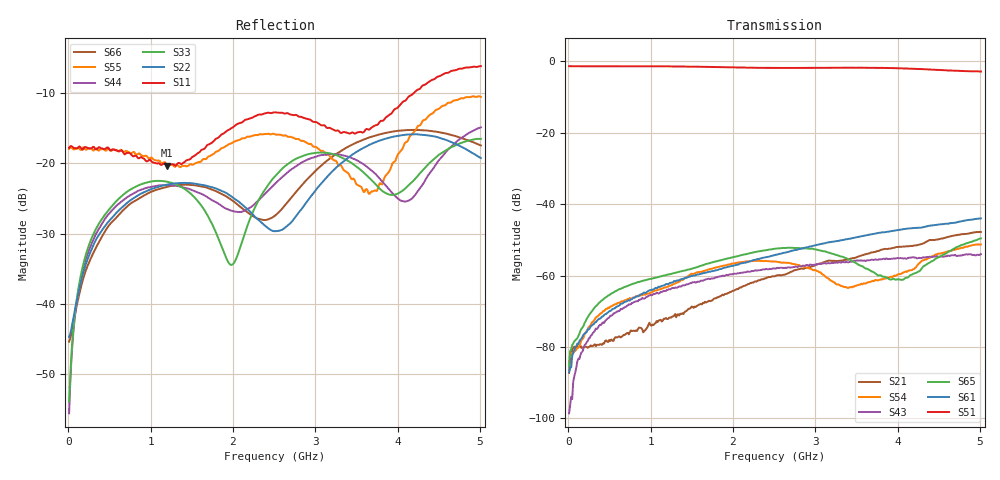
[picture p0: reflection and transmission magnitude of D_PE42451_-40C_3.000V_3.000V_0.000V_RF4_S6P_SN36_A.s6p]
! Device ID: PE42451
! Serial: 36
! Insertion: A
! Temp: -40C
! VDD: 3.000
! Control_Hi: 100.000
! Control_Lo: 0.000
! Logic State: RF4
! Port 1: RFC
! Port 2: RF1
! Port 3: RF2
! Port 4: RF3
! Port 5: RF4
! Port 6: RF5
! V1 = 0.00
! V2 = 0.00
! V3 = 3.00
! V4 = 0.00
! IDD: 1.326950e-05
#  Hz  S  RI  R  50
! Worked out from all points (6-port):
!   401 points, 10 MHz to 5.01 GHz, reference 50 ohm
!   strongest paths, dB at 10 MHz, 1.26 GHz, 2.51 GHz, 3.76 GHz, 5.01 GHz:
!     S51: -1.3, -1.4, -1.8, -1.8, -2.8
!     S61: -87.0, -61.9, -54.3, -48.1, -44.0
!     S65: -85.4, -59.5, -52.5, -60.0, -49.6
!     S43: -98.6, -63.5, -58.1, -55.6, -54.0
!     S54: -84.4, -62.6, -56.1, -61.4, -51.3
!     S21: -87.3, -71.5, -60.2, -53.1, -47.8
!   lowest |S11| = -20.3 dB at 1.198 GHz (marker M1), VSWR 1.21, Z = 55.2 - j8.7 ohm
!   |S11| at or under -10 dB: start of sweep to 4.193 GHz
